FUNCTION "FC_PROG_WD" : VOID
TITLE =WORK DECKS
VERSION : 0.1


VAR_TEMP
  WD1_TEMP_IN_RANGE : BOOL ;
  WD2_TEMP_IN_RANGE : BOOL ;
  WD1_F_UP_PURGING_SP : S5TIME ;
  WD2_F_UP_PURGING_SP : S5TIME ;
  T_81CLT81_COOL_SWP : REAL ;
  T_81CLT81_HEAT_SWP : REAL ;
  T_82CLT81_COOL_SWP : REAL ;
  T_82CLT81_HEAT_SWP : REAL ;
  T_81CLT81_READY_LOW : REAL ;
  T_81CLT81_READY_HIGH : REAL ;
  T_82CLT81_READY_LOW : REAL ;
  T_82CLT81_READY_HIGH : REAL ;
END_VAR
BEGIN
NETWORK
TITLE =SET MODE WORK DECKS 1+2 ON
//
//************************* SET MODE OF WORK DECK'S ******************************
//
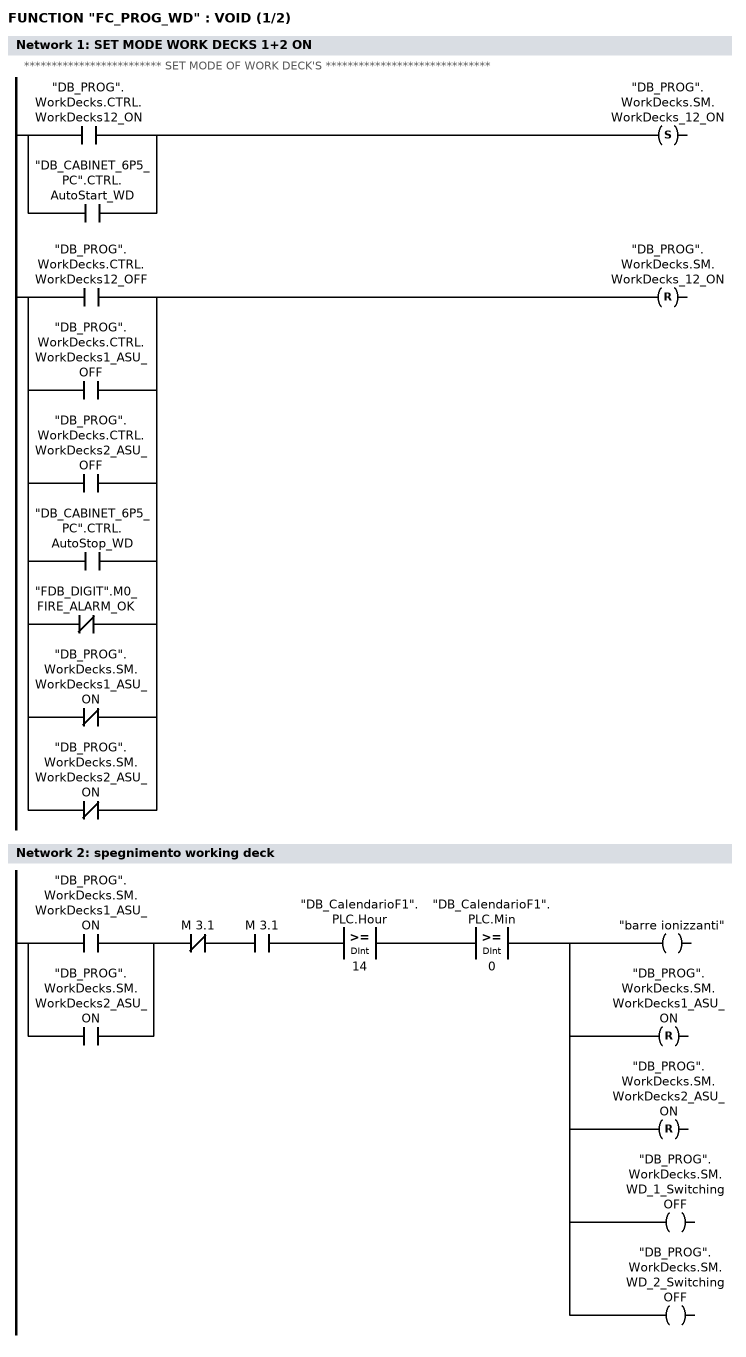
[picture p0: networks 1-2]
      U(    ;
      O     "DB_PROG".WorkDecks.CTRL.WorkDecks12_ON;
      O     "DB_CABINET_6P5_PC".CTRL.AutoStart_WD;
      )     ;
      S     "DB_PROG".WorkDecks.SM.WorkDecks_12_ON;
      U(    ;
      O     "DB_PROG".WorkDecks.CTRL.WorkDecks12_OFF;
      O     "DB_PROG".WorkDecks.CTRL.WorkDecks1_ASU_OFF;
      O     "DB_PROG".WorkDecks.CTRL.WorkDecks2_ASU_OFF;
      O     "DB_CABINET_6P5_PC".CTRL.AutoStop_WD;
      ON    "FDB_DIGIT".M0_FIRE_ALARM_OK;
      ON    "DB_PROG".WorkDecks.SM.WorkDecks1_ASU_ON;
      ON    "DB_PROG".WorkDecks.SM.WorkDecks2_ASU_ON;
      )     ;
      R     "DB_PROG".WorkDecks.SM.WorkDecks_12_ON;
      NOP   0;
NETWORK
TITLE =spegnimento working deck

      U(    ;
      O     "DB_PROG".WorkDecks.SM.WorkDecks1_ASU_ON;
      O     "DB_PROG".WorkDecks.SM.WorkDecks2_ASU_ON;
      )     ;
      UN    M      3.1;
      U     M      3.1;
      U(    ;
      L     "DB_CalendarioF1".PLC.Hour;
      L     14;
      >=D   ;
      )     ;
      U(    ;
      L     "DB_CalendarioF1".PLC.Min;
      L     0;
      >=D   ;
      )     ;
      =     "barre ionizzanti";
      R     "DB_PROG".WorkDecks.SM.WorkDecks1_ASU_ON;
      R     "DB_PROG".WorkDecks.SM.WorkDecks2_ASU_ON;
      =     "DB_PROG".WorkDecks.SM.WD_1_SwitchingOFF;
      =     "DB_PROG".WorkDecks.SM.WD_2_SwitchingOFF;
NETWORK
TITLE =SET MODE WORK DECKS 1 ON
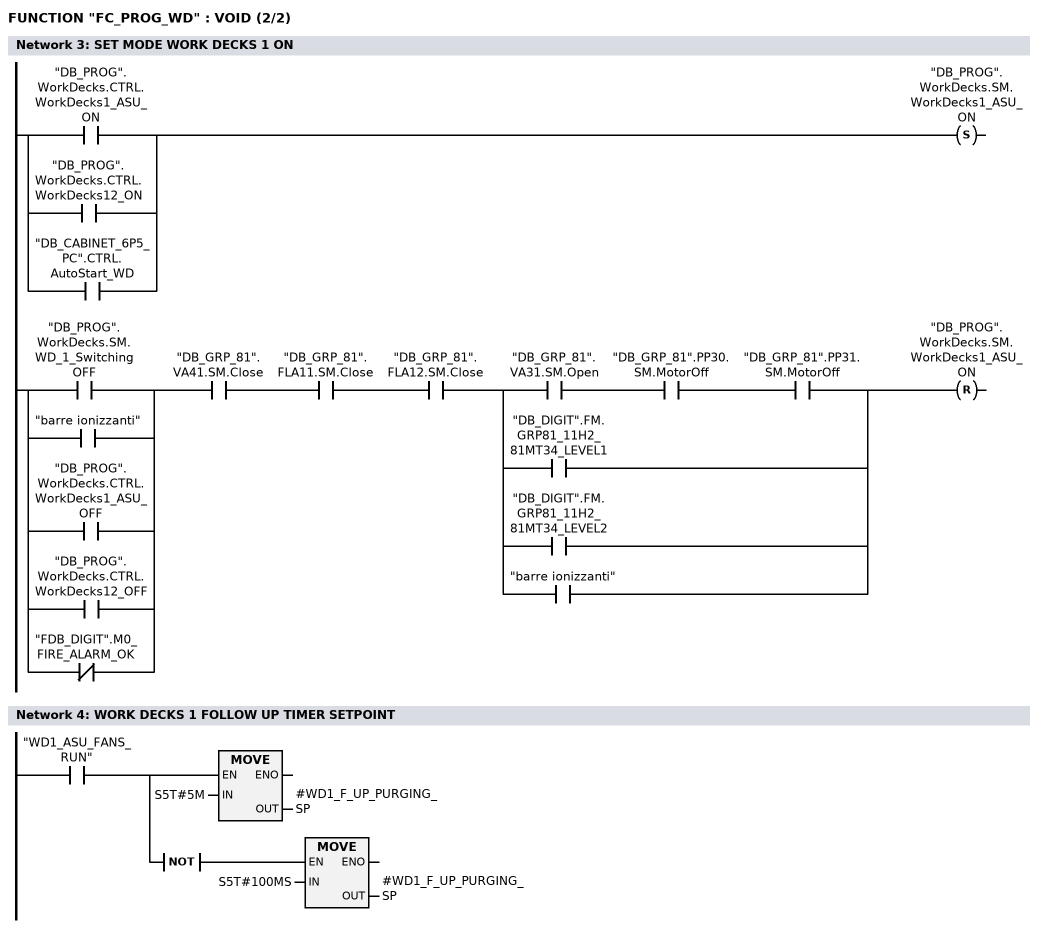
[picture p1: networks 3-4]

      U(    ;
      O     "DB_PROG".WorkDecks.CTRL.WorkDecks1_ASU_ON;
      O     "DB_PROG".WorkDecks.CTRL.WorkDecks12_ON;
      O     "DB_CABINET_6P5_PC".CTRL.AutoStart_WD;
      )     ;
      S     "DB_PROG".WorkDecks.SM.WorkDecks1_ASU_ON;
      U(    ;
      O     "DB_PROG".WorkDecks.SM.WD_1_SwitchingOFF;
      O     "barre ionizzanti";
      O     "DB_PROG".WorkDecks.CTRL.WorkDecks1_ASU_OFF;
      O     "DB_PROG".WorkDecks.CTRL.WorkDecks12_OFF;
      ON    "FDB_DIGIT".M0_FIRE_ALARM_OK;
      )     ;
      U     "DB_GRP_81".VA41.SM.Close;
      U     "DB_GRP_81".FLA11.SM.Close;
      U     "DB_GRP_81".FLA12.SM.Close;
      U(    ;
      U     "DB_GRP_81".VA31.SM.Open;
      U     "DB_GRP_81".PP30.SM.MotorOff;
      U     "DB_GRP_81".PP31.SM.MotorOff;
      O     "DB_DIGIT".FM.GRP81_11H2_81MT34_LEVEL1;
      O     "DB_DIGIT".FM.GRP81_11H2_81MT34_LEVEL2;
      O     "barre ionizzanti";
      )     ;
      R     "DB_PROG".WorkDecks.SM.WorkDecks1_ASU_ON;
      NOP   0;
NETWORK
TITLE =WORK DECKS 1 FOLLOW UP TIMER SETPOINT

      U     "WD1_ASU_FANS_RUN";
      =     L     38.0;
      U     L     38.0;
      SPBNB _001;
      L     S5T#5M;
      T     #WD1_F_UP_PURGING_SP;
_001: NOP   0;
      U     L     38.0;
      NOT   ;
      SPBNB _002;
      L     S5T#100MS;
      T     #WD1_F_UP_PURGING_SP;
_002: NOP   0;
NETWORK
TITLE =SET MODE WORK DECKS 1 SWITCHING OFF
//
//
      U(    ;
      U(    ;
      O     "DB_PROG".WorkDecks.CTRL.WorkDecks1_ASU_OFF;
      O     "barre ionizzanti";
      ON    "DB_PROG".WorkDecks.SM.WorkDecks_12_ON;
      ON    "FDB_DIGIT".M0_FIRE_ALARM_OK;
      )     ;
      U     "DB_CABINET_6P5_R11".SM.CtrlVoltageON;
      S     "DB_PROG".WorkDecks.SM.WD_1_SwitchingOFF;
      U(    ;
      U     "DB_GRP_81".VA41.SM.Close;
      U     "DB_GRP_81".FLA11.SM.Close;
      U     "DB_GRP_81".FLA12.SM.Close;
      U(    ;
      U     "DB_GRP_81".VA31.SM.Open;
      U     "DB_GRP_81".PP30.SM.MotorOff;
      U     "DB_GRP_81".PP31.SM.MotorOff;
      O     "DB_DIGIT".FM.GRP81_11H2_81MT34_LEVEL1;
      O     "DB_DIGIT".FM.GRP81_11H2_81MT34_LEVEL2;
      )     ;
      O     "DB_PROG".WorkDecks.CTRL.WorkDecks1_ASU_ON;
      O     "DB_PROG".WorkDecks.SM.WorkDecks_12_ON;
      )     ;
      R     "DB_PROG".WorkDecks.SM.WD_1_SwitchingOFF;
      U     "DB_PROG".WorkDecks.SM.WD_1_SwitchingOFF;
      )     ;
      L     #WD1_F_UP_PURGING_SP;
      SE    "T_FOLLOW_UP_PURGING_WD1";
      U(    ;
      O     "DB_PROG".WorkDecks.CTRL.WorkDecks1_ASU_ON;
      O     "DB_PROG".WorkDecks.SM.WorkDecks_12_ON;
      )     ;
      R     "T_FOLLOW_UP_PURGING_WD1";
      NOP   0;
      NOP   0;
      NOP   0;
NETWORK
TITLE =SET MODE WORK DECKS 2 ON
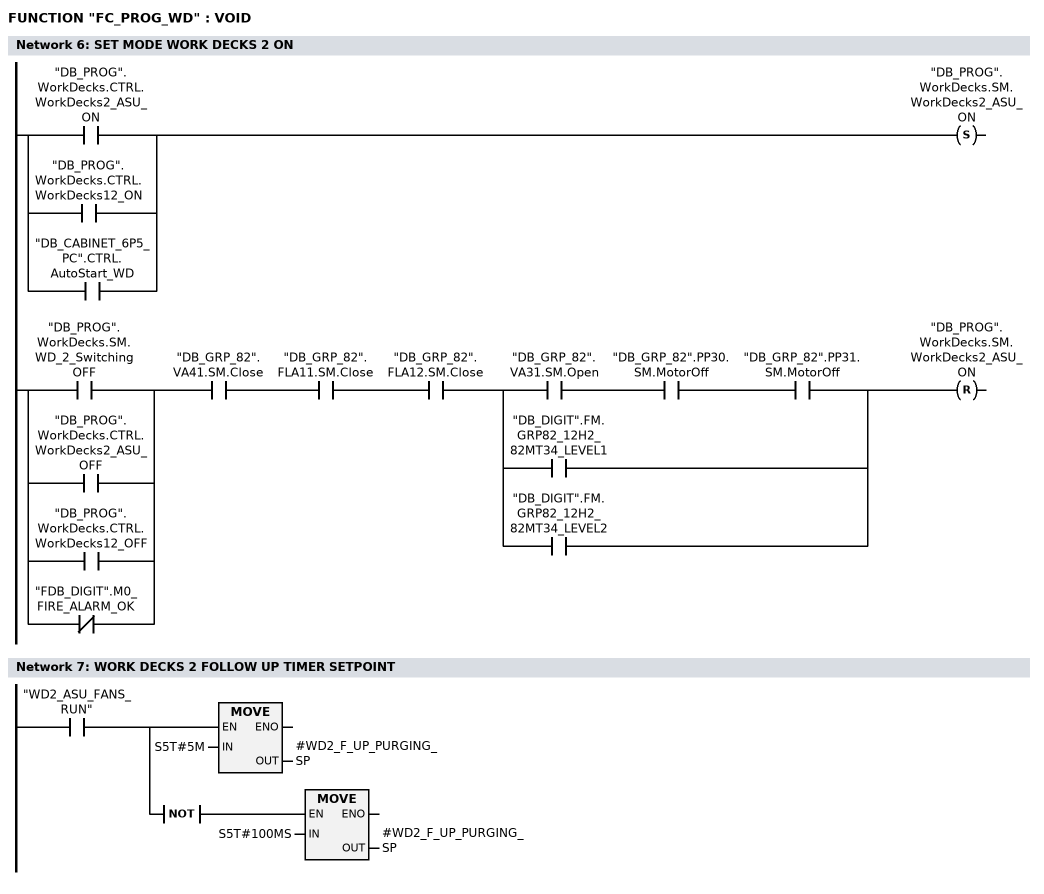
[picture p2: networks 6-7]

      U(    ;
      O     "DB_PROG".WorkDecks.CTRL.WorkDecks2_ASU_ON;
      O     "DB_PROG".WorkDecks.CTRL.WorkDecks12_ON;
      O     "DB_CABINET_6P5_PC".CTRL.AutoStart_WD;
      )     ;
      S     "DB_PROG".WorkDecks.SM.WorkDecks2_ASU_ON;
      U(    ;
      O     "DB_PROG".WorkDecks.SM.WD_2_SwitchingOFF;
      O     "DB_PROG".WorkDecks.CTRL.WorkDecks2_ASU_OFF;
      O     "DB_PROG".WorkDecks.CTRL.WorkDecks12_OFF;
      ON    "FDB_DIGIT".M0_FIRE_ALARM_OK;
      )     ;
      U     "DB_GRP_82".VA41.SM.Close;
      U     "DB_GRP_82".FLA11.SM.Close;
      U     "DB_GRP_82".FLA12.SM.Close;
      U(    ;
      U     "DB_GRP_82".VA31.SM.Open;
      U     "DB_GRP_82".PP30.SM.MotorOff;
      U     "DB_GRP_82".PP31.SM.MotorOff;
      O     "DB_DIGIT".FM.GRP82_12H2_82MT34_LEVEL1;
      O     "DB_DIGIT".FM.GRP82_12H2_82MT34_LEVEL2;
      )     ;
      R     "DB_PROG".WorkDecks.SM.WorkDecks2_ASU_ON;
      NOP   0;
NETWORK
TITLE =WORK DECKS 2 FOLLOW UP TIMER SETPOINT

      U     "WD2_ASU_FANS_RUN";
      =     L     38.0;
      U     L     38.0;
      SPBNB _003;
      L     S5T#5M;
      T     #WD2_F_UP_PURGING_SP;
_003: NOP   0;
      U     L     38.0;
      NOT   ;
      SPBNB _004;
      L     S5T#100MS;
      T     #WD2_F_UP_PURGING_SP;
_004: NOP   0;
NETWORK
TITLE =SET MODE WORK DECKS 2 SWITCHING OFF

      U(    ;
      U(    ;
      O     "DB_PROG".WorkDecks.CTRL.WorkDecks2_ASU_OFF;
      ON    "DB_PROG".WorkDecks.SM.WorkDecks_12_ON;
      ON    "FDB_DIGIT".M0_FIRE_ALARM_OK;
      )     ;
      U     "DB_CABINET_6P5_R12".SM.CtrlVoltageON;
      S     "DB_PROG".WorkDecks.SM.WD_2_SwitchingOFF;
      U(    ;
      U     "DB_GRP_82".VA41.SM.Close;
      U     "DB_GRP_82".FLA11.SM.Close;
      U     "DB_GRP_82".FLA12.SM.Close;
      U(    ;
      U     "DB_GRP_82".VA31.SM.Open;
      U     "DB_GRP_82".PP30.SM.MotorOff;
      U     "DB_GRP_82".PP31.SM.MotorOff;
      O     "DB_DIGIT".FM.GRP82_12H2_82MT34_LEVEL1;
      O     "DB_DIGIT".FM.GRP82_12H2_82MT34_LEVEL2;
      )     ;
      O     "DB_PROG".WorkDecks.CTRL.WorkDecks2_ASU_ON;
      O     "DB_PROG".WorkDecks.SM.WorkDecks_12_ON;
      )     ;
      R     "DB_PROG".WorkDecks.SM.WD_2_SwitchingOFF;
      U     "DB_PROG".WorkDecks.SM.WD_2_SwitchingOFF;
      )     ;
      L     #WD2_F_UP_PURGING_SP;
      SE    "T_FOLLOW_UP_PURGING_WD2";
      U(    ;
      O     "DB_PROG".WorkDecks.CTRL.WorkDecks2_ASU_ON;
      O     "DB_PROG".WorkDecks.SM.WorkDecks_12_ON;
      )     ;
      R     "T_FOLLOW_UP_PURGING_WD2";
      NOP   0;
      NOP   0;
      NOP   0;
NETWORK
TITLE =SET MODE VENTILATION SKID OFF-CLEANING ON
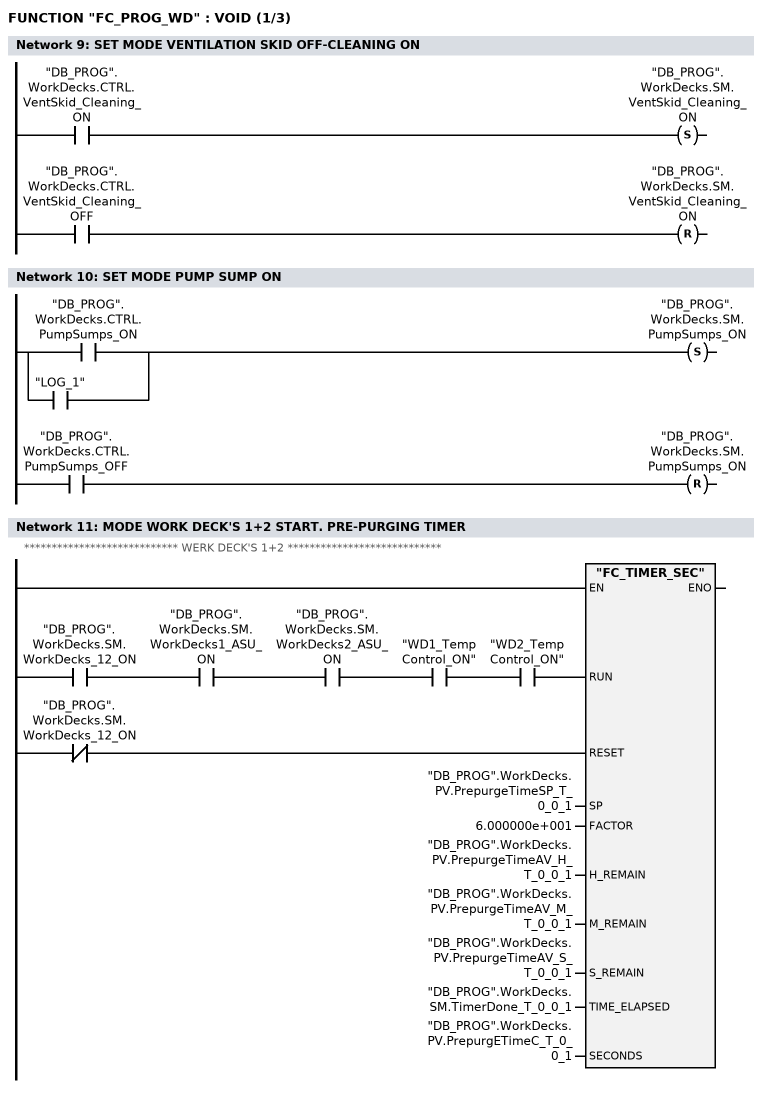
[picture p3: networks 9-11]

      U     "DB_PROG".WorkDecks.CTRL.VentSkid_Cleaning_ON;
      S     "DB_PROG".WorkDecks.SM.VentSkid_Cleaning_ON;
      U     "DB_PROG".WorkDecks.CTRL.VentSkid_Cleaning_OFF;
      R     "DB_PROG".WorkDecks.SM.VentSkid_Cleaning_ON;
      NOP   0;
NETWORK
TITLE =SET MODE PUMP SUMP ON

      U(    ;
      O     "DB_PROG".WorkDecks.CTRL.PumpSumps_ON;
      O     "LOG_1";
      )     ;
      S     "DB_PROG".WorkDecks.SM.PumpSumps_ON;
      U     "DB_PROG".WorkDecks.CTRL.PumpSumps_OFF;
      R     "DB_PROG".WorkDecks.SM.PumpSumps_ON;
      NOP   0;
NETWORK
TITLE =MODE WORK DECK'S 1+2 START. PRE-PURGING TIMER
//
//**************************** WERK DECK'S 1+2 ****************************
//
      U     "DB_PROG".WorkDecks.SM.WorkDecks_12_ON;
      U     "DB_PROG".WorkDecks.SM.WorkDecks1_ASU_ON;
      U     "DB_PROG".WorkDecks.SM.WorkDecks2_ASU_ON;
      U     "WD1_TempControl_ON";
      U     "WD2_TempControl_ON";
      =     L     38.0;
      BLD   103;
      UN    "DB_PROG".WorkDecks.SM.WorkDecks_12_ON;
      =     L     38.1;
      BLD   103;
      CALL "FC_TIMER_SEC" (
           RUN                      := L     38.0,
           RESET                    := L     38.1,
           SP                       := "DB_PROG".WorkDecks.PV.PrepurgeTimeSP_T_0_0_1,
           FACTOR                   := 6.000000e+001,
           H_REMAIN                 := "DB_PROG".WorkDecks.PV.PrepurgeTimeAV_H_T_0_0_1,
           M_REMAIN                 := "DB_PROG".WorkDecks.PV.PrepurgeTimeAV_M_T_0_0_1,
           S_REMAIN                 := "DB_PROG".WorkDecks.PV.PrepurgeTimeAV_S_T_0_0_1,
           TIME_ELAPSED             := "DB_PROG".WorkDecks.SM.TimerDone_T_0_0_1,
           SECONDS                  := "DB_PROG".WorkDecks.PV.PrepurgETimeC_T_0_0_1);
      NOP   0;
NETWORK
TITLE =MODE WORK DECK'S 1 START. PRE-PURGING TIMER
//
//**************************** WERK DECK'S 1 ****************************
//
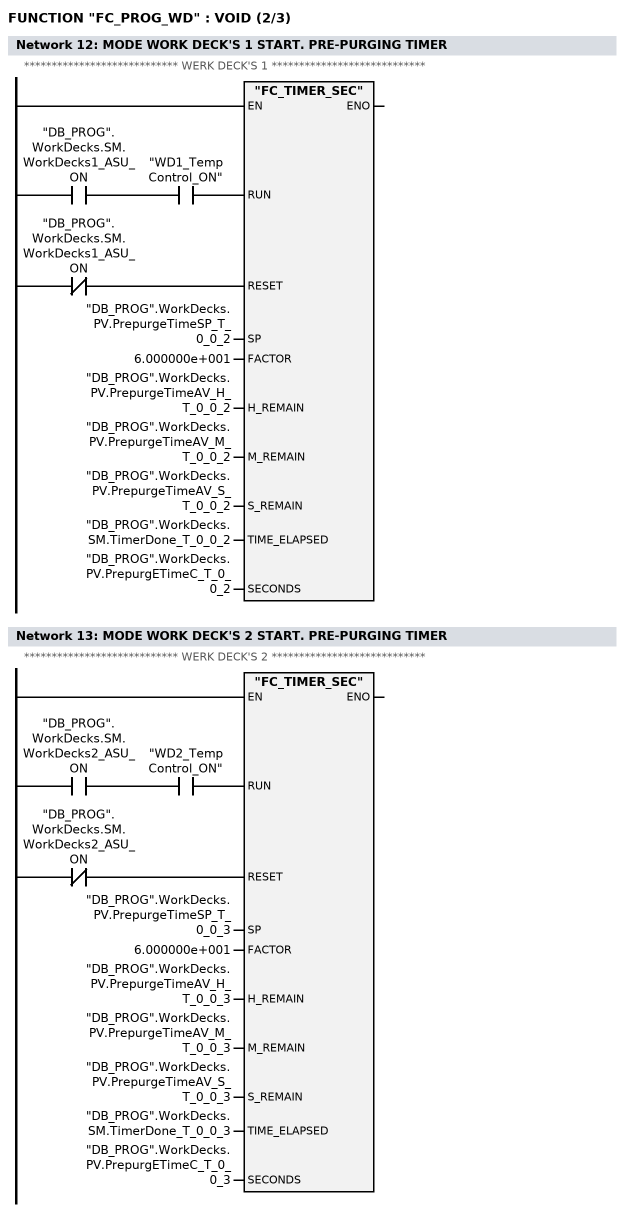
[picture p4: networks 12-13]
      U     "DB_PROG".WorkDecks.SM.WorkDecks1_ASU_ON;
      U     "WD1_TempControl_ON";
      =     L     38.0;
      BLD   103;
      UN    "DB_PROG".WorkDecks.SM.WorkDecks1_ASU_ON;
      =     L     38.1;
      BLD   103;
      CALL "FC_TIMER_SEC" (
           RUN                      := L     38.0,
           RESET                    := L     38.1,
           SP                       := "DB_PROG".WorkDecks.PV.PrepurgeTimeSP_T_0_0_2,
           FACTOR                   := 6.000000e+001,
           H_REMAIN                 := "DB_PROG".WorkDecks.PV.PrepurgeTimeAV_H_T_0_0_2,
           M_REMAIN                 := "DB_PROG".WorkDecks.PV.PrepurgeTimeAV_M_T_0_0_2,
           S_REMAIN                 := "DB_PROG".WorkDecks.PV.PrepurgeTimeAV_S_T_0_0_2,
           TIME_ELAPSED             := "DB_PROG".WorkDecks.SM.TimerDone_T_0_0_2,
           SECONDS                  := "DB_PROG".WorkDecks.PV.PrepurgETimeC_T_0_0_2);
      NOP   0;
NETWORK
TITLE =MODE WORK DECK'S 2 START. PRE-PURGING TIMER
//
//**************************** WERK DECK'S 2 ****************************
//
      U     "DB_PROG".WorkDecks.SM.WorkDecks2_ASU_ON;
      U     "WD2_TempControl_ON";
      =     L     38.0;
      BLD   103;
      UN    "DB_PROG".WorkDecks.SM.WorkDecks2_ASU_ON;
      =     L     38.1;
      BLD   103;
      CALL "FC_TIMER_SEC" (
           RUN                      := L     38.0,
           RESET                    := L     38.1,
           SP                       := "DB_PROG".WorkDecks.PV.PrepurgeTimeSP_T_0_0_3,
           FACTOR                   := 6.000000e+001,
           H_REMAIN                 := "DB_PROG".WorkDecks.PV.PrepurgeTimeAV_H_T_0_0_3,
           M_REMAIN                 := "DB_PROG".WorkDecks.PV.PrepurgeTimeAV_M_T_0_0_3,
           S_REMAIN                 := "DB_PROG".WorkDecks.PV.PrepurgeTimeAV_S_T_0_0_3,
           TIME_ELAPSED             := "DB_PROG".WorkDecks.SM.TimerDone_T_0_0_3,
           SECONDS                  := "DB_PROG".WorkDecks.PV.PrepurgETimeC_T_0_0_3);
      NOP   0;
NETWORK
TITLE =MODE WORK DECK'S OFF-LINE SKID CLEANING START. PRE-PURGING TIMER
//
//****************** WORK DECK'S OFF-LINE SKID CLEANING *******************
//
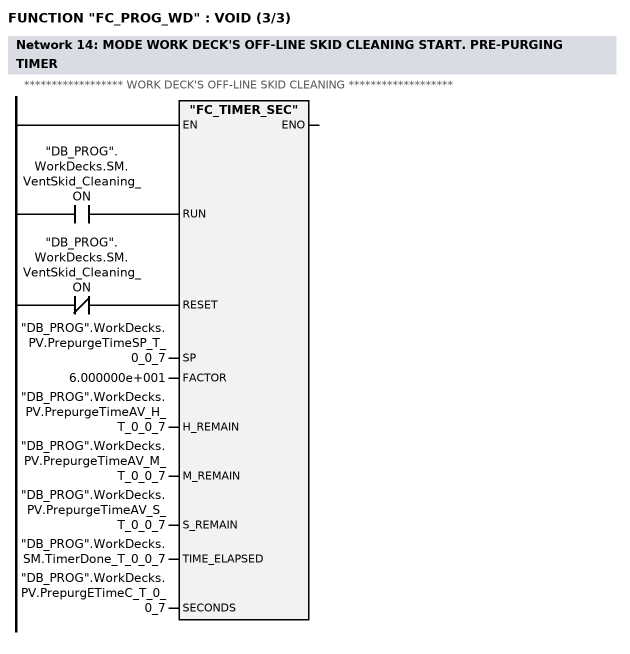
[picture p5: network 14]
      U     "DB_PROG".WorkDecks.SM.VentSkid_Cleaning_ON;
      =     L     38.0;
      BLD   103;
      UN    "DB_PROG".WorkDecks.SM.VentSkid_Cleaning_ON;
      =     L     38.1;
      BLD   103;
      CALL "FC_TIMER_SEC" (
           RUN                      := L     38.0,
           RESET                    := L     38.1,
           SP                       := "DB_PROG".WorkDecks.PV.PrepurgeTimeSP_T_0_0_7,
           FACTOR                   := 6.000000e+001,
           H_REMAIN                 := "DB_PROG".WorkDecks.PV.PrepurgeTimeAV_H_T_0_0_7,
           M_REMAIN                 := "DB_PROG".WorkDecks.PV.PrepurgeTimeAV_M_T_0_0_7,
           S_REMAIN                 := "DB_PROG".WorkDecks.PV.PrepurgeTimeAV_S_T_0_0_7,
           TIME_ELAPSED             := "DB_PROG".WorkDecks.SM.TimerDone_T_0_0_7,
           SECONDS                  := "DB_PROG".WorkDecks.PV.PrepurgETimeC_T_0_0_7);
      NOP   0;
NETWORK
TITLE =MODE START WORK DECK'S 1
//
//**************** START SEQUENTION WORK DECK'S 1 ******************************
//
      U(    ;
      U(    ;
      O     "DB_PROG".WorkDecks.CTRL.WorkDecks1_ASU_ON;
      O     "DB_PROG".WorkDecks.SM.WorkDecks_12_ON;
      )     ;
      S     "WD1_ASU_StartPump";
      U     "WD1_StartFinished";
      R     "WD1_ASU_StartPump";
      U     "WD1_ASU_StartPump";
      )     ;
      L     S5T#5M;
      SE    "T_2_0_10";
      NOP   0;
      NOP   0;
      NOP   0;
      NOP   0;
NETWORK
TITLE =WORK DECKS #1 DELAY STOP PUMP =81PP31 ASU WD1, WHEN TEMP>TEMP_SP
//
//
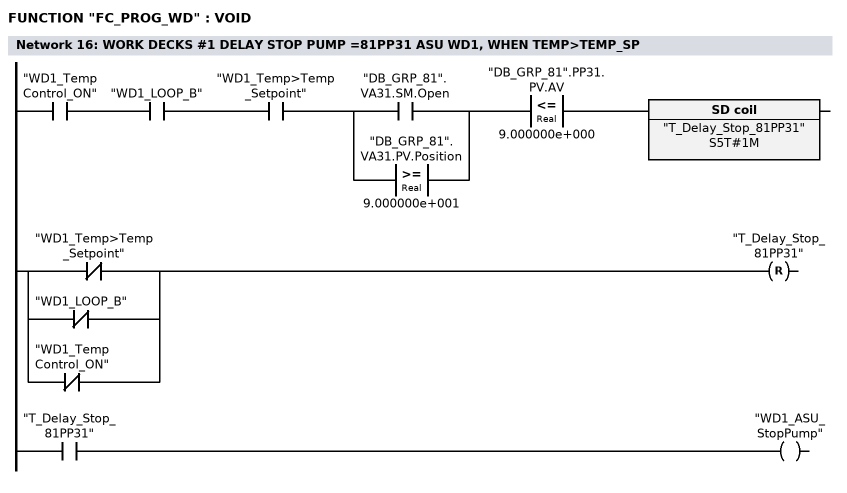
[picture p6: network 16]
      U     "WD1_TempControl_ON";
      U     "WD1_LOOP_B";
      U     "WD1_Temp>Temp_Setpoint";
      U(    ;
      O     "DB_GRP_81".VA31.SM.Open;
      O(    ;
      L     "DB_GRP_81".VA31.PV.Position;
      L     9.000000e+001;
      >=R   ;
      )     ;
      )     ;
      U(    ;
      L     "DB_GRP_81".PP31.PV.AV;
      L     9.000000e+000;
      <=R   ;
      )     ;
      L     S5T#1M;
      SE    "T_Delay_Stop_81PP31";
      U(    ;
      ON    "WD1_Temp>Temp_Setpoint";
      ON    "WD1_LOOP_B";
      ON    "WD1_TempControl_ON";
      )     ;
      R     "T_Delay_Stop_81PP31";
      NOP   0;
      NOP   0;
      U     "T_Delay_Stop_81PP31";
      =     "WD1_ASU_StopPump";
NETWORK
TITLE =START FLAPS ASU WD 1

      U     "DB_PROG".WorkDecks.SM.WorkDecks1_ASU_ON;
      U(    ;
      O     "T_2_0_10";
      O     "WD1_StartFinished";
      )     ;
      UN    "DB_MULFUNCTION".SM.WD1_MALFUNCTION_STOP;
      S     "WD1_OpenFlaps";
      U(    ;
      U(    ;
      U     "DB_PROG".WorkDecks.SM.WD_1_SwitchingOFF;
      U     "DB_GRP_81".FAN71.SM.MotorOff;
      U(    ;
      U     "DB_GRP_81".FAN01.SM.MotorOff;
      U     "DB_GRP_82".FAN02.SM.MotorOff;
      ON    "DB_PROG".WorkDecks.SM.WorkDecks_12_ON;
      )     ;
      O     "DB_DIGIT".FM.GRP81_11H2_81MT34_LEVEL2;
      )     ;
      L     S5T#3M;
      SE    "T_5_0_2";
      NOP   0;
      NOP   0;
      NOP   0;
      U     "T_5_0_2";
      )     ;
      R     "WD1_OpenFlaps";
      NOP   0;
NETWORK
TITLE =VENTILATION WORK DECK'S 1 RUNNING (SIGNAL TO SHOP)
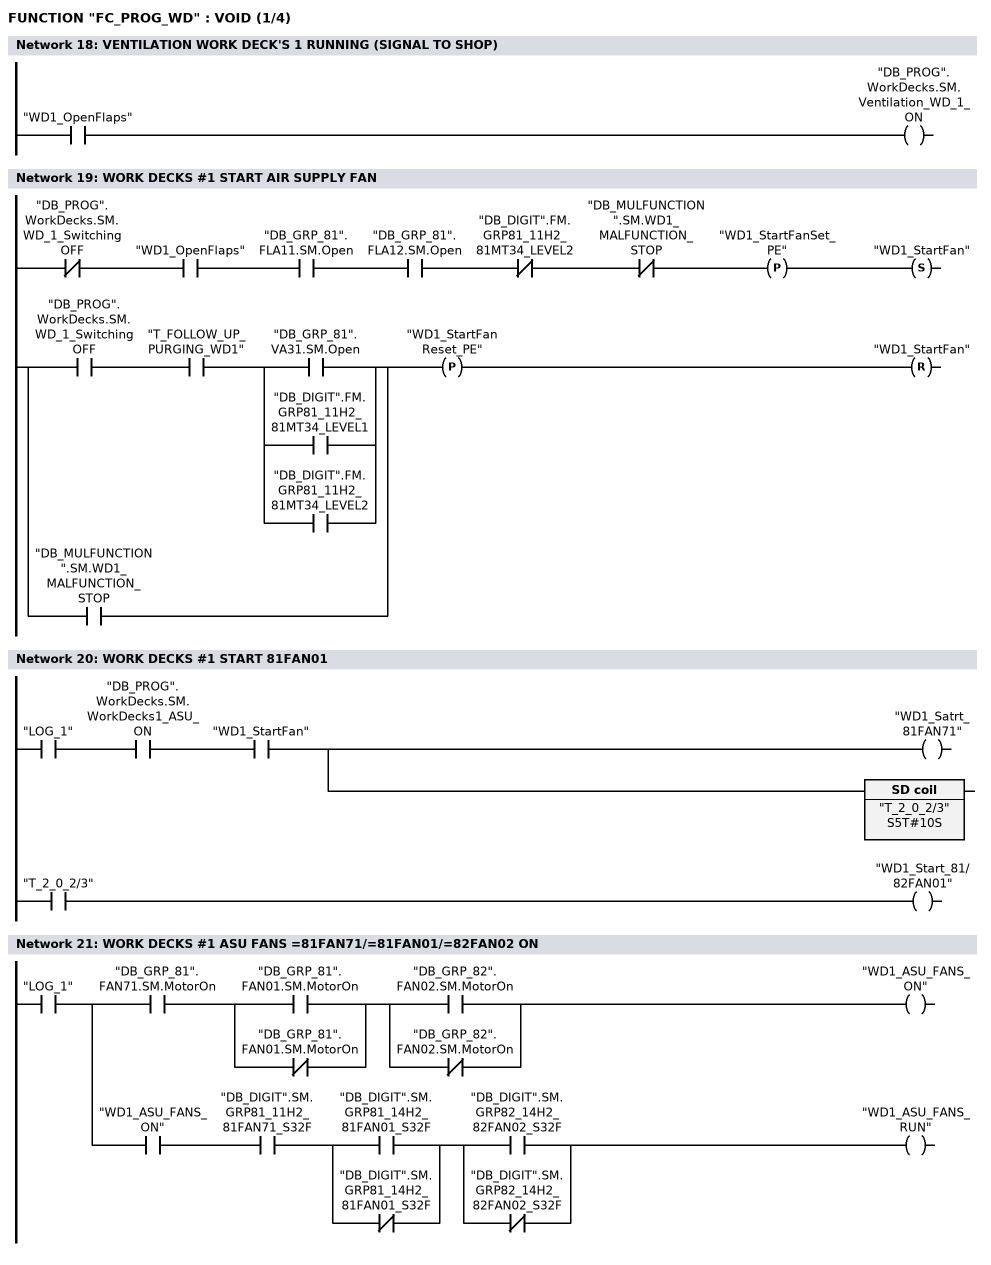
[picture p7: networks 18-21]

      U     "WD1_OpenFlaps";
      =     "DB_PROG".WorkDecks.SM.Ventilation_WD_1_ON;
NETWORK
TITLE =WORK DECKS #1 START AIR SUPPLY FAN

      UN    "DB_PROG".WorkDecks.SM.WD_1_SwitchingOFF;
      U     "WD1_OpenFlaps";
      U     "DB_GRP_81".FLA11.SM.Open;
      U     "DB_GRP_81".FLA12.SM.Open;
      UN    "DB_DIGIT".FM.GRP81_11H2_81MT34_LEVEL2;
      UN    "DB_MULFUNCTION".SM.WD1_MALFUNCTION_STOP;
      FP    "WD1_StartFanSet_PE";
      S     "WD1_StartFan";
      U(    ;
      U     "DB_PROG".WorkDecks.SM.WD_1_SwitchingOFF;
      U     "T_FOLLOW_UP_PURGING_WD1";
      U(    ;
      O     "DB_GRP_81".VA31.SM.Open;
      O     "DB_DIGIT".FM.GRP81_11H2_81MT34_LEVEL1;
      O     "DB_DIGIT".FM.GRP81_11H2_81MT34_LEVEL2;
      )     ;
      O     "DB_MULFUNCTION".SM.WD1_MALFUNCTION_STOP;
      )     ;
      FP    "WD1_StartFanReset_PE";
      R     "WD1_StartFan";
      NOP   0;
NETWORK
TITLE =WORK DECKS #1 START 81FAN01

      U     "LOG_1";
      U     "DB_PROG".WorkDecks.SM.WorkDecks1_ASU_ON;
      U     "WD1_StartFan";
      =     L     38.0;
      U     L     38.0;
      BLD   102;
      =     "WD1_Satrt_81FAN71";
      U     L     38.0;
      L     S5T#10S;
      SE    "T_2_0_2/3";
      NOP   0;
      NOP   0;
      NOP   0;
      U     "T_2_0_2/3";
      =     "WD1_Start_81/82FAN01";
NETWORK
TITLE =WORK DECKS #1 ASU FANS =81FAN71/=81FAN01/=82FAN02 ON

      U     "LOG_1";
      =     L     38.0;
      U     L     38.0;
      U     "DB_GRP_81".FAN71.SM.MotorOn;
      U(    ;
      O     "DB_GRP_81".FAN01.SM.MotorOn;
      ON    "DB_GRP_81".FAN01.SM.MotorOn;
      )     ;
      U(    ;
      O     "DB_GRP_82".FAN02.SM.MotorOn;
      ON    "DB_GRP_82".FAN02.SM.MotorOn;
      )     ;
      =     "WD1_ASU_FANS_ON";
      U     L     38.0;
      U     "WD1_ASU_FANS_ON";
      U     "DB_DIGIT".SM.GRP81_11H2_81FAN71_S32F;
      U(    ;
      O     "DB_DIGIT".SM.GRP81_14H2_81FAN01_S32F;
      ON    "DB_DIGIT".SM.GRP81_14H2_81FAN01_S32F;
      )     ;
      U(    ;
      O     "DB_DIGIT".SM.GRP82_14H2_82FAN02_S32F;
      ON    "DB_DIGIT".SM.GRP82_14H2_82FAN02_S32F;
      )     ;
      =     "WD1_ASU_FANS_RUN";
NETWORK
TITLE =WORK DECKS #1 TEMPERATURE CONTROL ON (PAP 1.5.1)
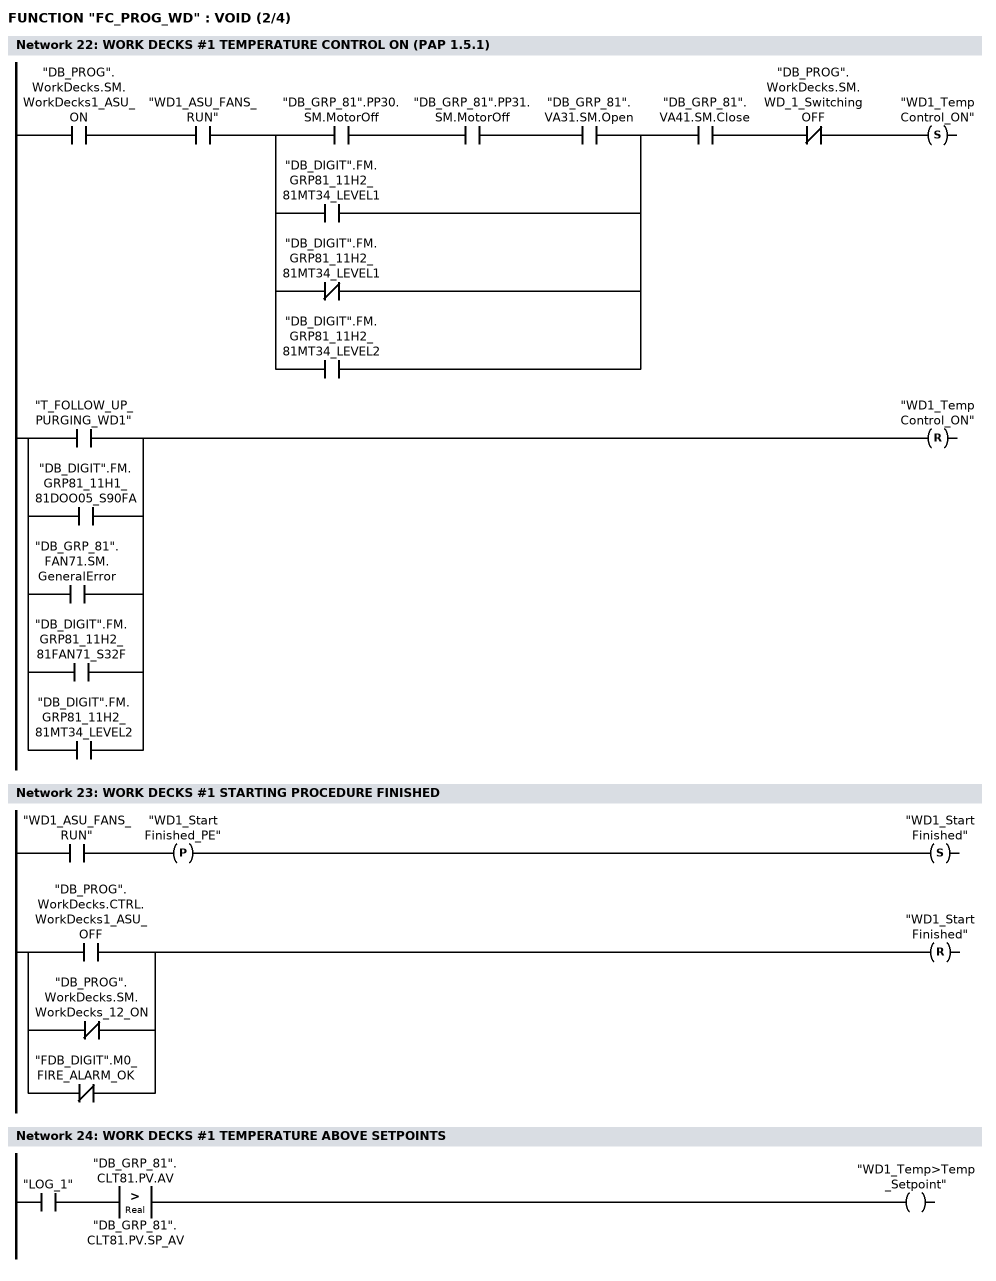
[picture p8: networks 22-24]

      U     "DB_PROG".WorkDecks.SM.WorkDecks1_ASU_ON;
      U     "WD1_ASU_FANS_RUN";
      U(    ;
      U     "DB_GRP_81".PP30.SM.MotorOff;
      U     "DB_GRP_81".PP31.SM.MotorOff;
      U     "DB_GRP_81".VA31.SM.Open;
      O     "DB_DIGIT".FM.GRP81_11H2_81MT34_LEVEL1;
      ON    "DB_DIGIT".FM.GRP81_11H2_81MT34_LEVEL1;
      O     "DB_DIGIT".FM.GRP81_11H2_81MT34_LEVEL2;
      )     ;
      U     "DB_GRP_81".VA41.SM.Close;
      UN    "DB_PROG".WorkDecks.SM.WD_1_SwitchingOFF;
      S     "WD1_TempControl_ON";
      U(    ;
      O     "T_FOLLOW_UP_PURGING_WD1";
      O     "DB_DIGIT".FM.GRP81_11H1_81DOO05_S90FA;
      O     "DB_GRP_81".FAN71.SM.GeneralError;
      O     "DB_DIGIT".FM.GRP81_11H2_81FAN71_S32F;
      O     "DB_DIGIT".FM.GRP81_11H2_81MT34_LEVEL2;
      )     ;
      R     "WD1_TempControl_ON";
      NOP   0;
NETWORK
TITLE =WORK DECKS #1 STARTING PROCEDURE FINISHED

      U     "WD1_ASU_FANS_RUN";
      FP    "WD1_StartFinished_PE";
      S     "WD1_StartFinished";
      U(    ;
      O     "DB_PROG".WorkDecks.CTRL.WorkDecks1_ASU_OFF;
      ON    "DB_PROG".WorkDecks.SM.WorkDecks_12_ON;
      ON    "FDB_DIGIT".M0_FIRE_ALARM_OK;
      )     ;
      R     "WD1_StartFinished";
      NOP   0;
NETWORK
TITLE =WORK DECKS #1 TEMPERATURE ABOVE SETPOINTS

      U     "LOG_1";
      U(    ;
      L     "DB_GRP_81".CLT81.PV.AV;
      L     "DB_GRP_81".CLT81.PV.SP_AV;
      >R    ;
      )     ;
      =     "WD1_Temp>Temp_Setpoint";
NETWORK
TITLE =WORK DECKS #1 SET SWITCHING POINTS
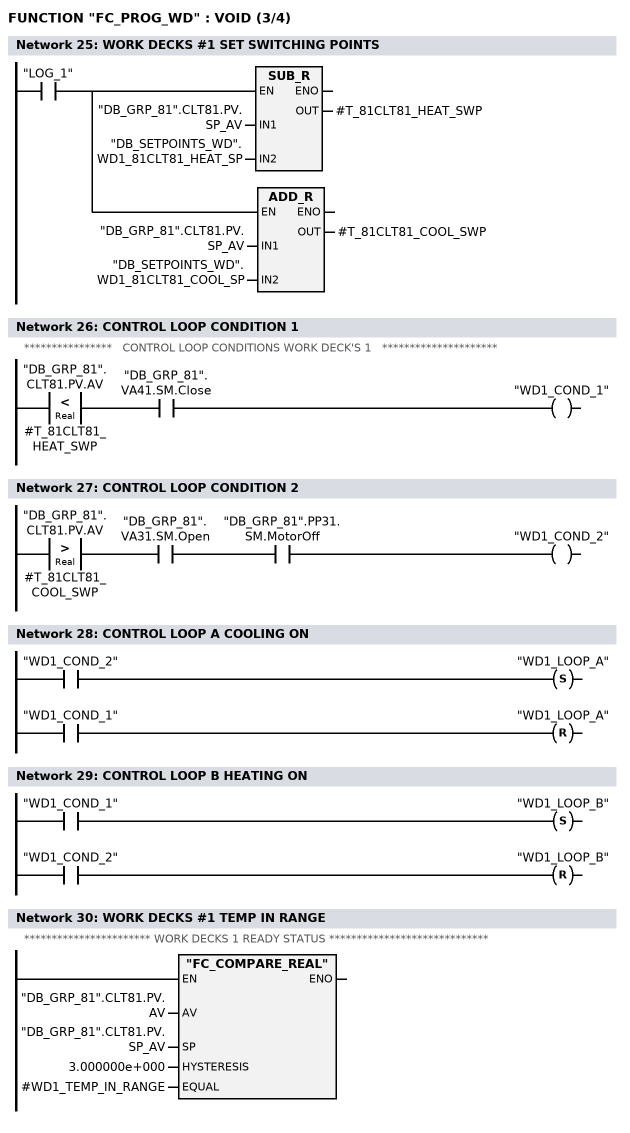
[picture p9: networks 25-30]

      U     "LOG_1";
      =     L     38.0;
      U     L     38.0;
      SPBNB _005;
      L     "DB_GRP_81".CLT81.PV.SP_AV;
      L     "DB_SETPOINTS_WD".WD1_81CLT81_HEAT_SP;
      -R    ;
      T     #T_81CLT81_HEAT_SWP;
_005: NOP   0;
      U     L     38.0;
      SPBNB _006;
      L     "DB_GRP_81".CLT81.PV.SP_AV;
      L     "DB_SETPOINTS_WD".WD1_81CLT81_COOL_SP;
      +R    ;
      T     #T_81CLT81_COOL_SWP;
_006: NOP   0;
NETWORK
TITLE =CONTROL LOOP CONDITION 1
//
//****************   CONTROL LOOP CONDITIONS WORK DECK'S 1   *********************
//
//
      U(    ;
      L     "DB_GRP_81".CLT81.PV.AV;
      L     #T_81CLT81_HEAT_SWP;
      <R    ;
      )     ;
      U     "DB_GRP_81".VA41.SM.Close;
      =     "WD1_COND_1";
NETWORK
TITLE =CONTROL LOOP CONDITION 2

      U(    ;
      L     "DB_GRP_81".CLT81.PV.AV;
      L     #T_81CLT81_COOL_SWP;
      >R    ;
      )     ;
      U     "DB_GRP_81".VA31.SM.Open;
      U     "DB_GRP_81".PP31.SM.MotorOff;
      =     "WD1_COND_2";
NETWORK
TITLE =CONTROL LOOP A COOLING ON

      U     "WD1_COND_2";
      S     "WD1_LOOP_A";
      U     "WD1_COND_1";
      R     "WD1_LOOP_A";
      NOP   0;
NETWORK
TITLE =CONTROL LOOP B HEATING ON

      U     "WD1_COND_1";
      S     "WD1_LOOP_B";
      U     "WD1_COND_2";
      R     "WD1_LOOP_B";
      NOP   0;
NETWORK
TITLE =WORK DECKS #1 TEMP IN RANGE
//
//*********************** WORK DECKS 1 READY STATUS *****************************
//
      CALL "FC_COMPARE_REAL" (
           AV                       := "DB_GRP_81".CLT81.PV.AV,
           SP                       := "DB_GRP_81".CLT81.PV.SP_AV,
           HYSTERESIS               := 3.000000e+000,
           EQUAL                    := #WD1_TEMP_IN_RANGE);
      NOP   0;
NETWORK
TITLE =WORK DECKS #1 WINDOW TO READY STATUS IN POWER SAVING MODE 2
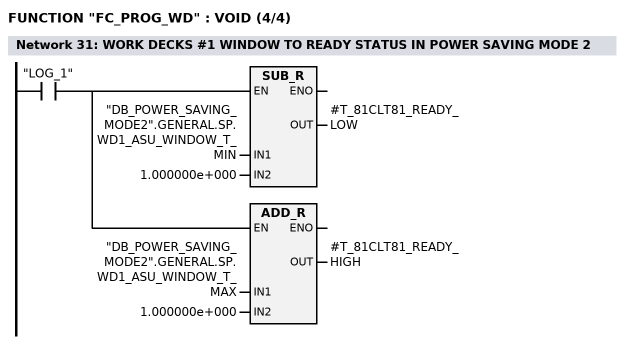
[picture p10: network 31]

      U     "LOG_1";
      =     L     38.0;
      U     L     38.0;
      SPBNB _007;
      L     "DB_POWER_SAVING_MODE2".GENERAL.SP.WD1_ASU_WINDOW_T_MIN;
      L     1.000000e+000;
      -R    ;
      T     #T_81CLT81_READY_LOW;
_007: NOP   0;
      U     L     38.0;
      SPBNB _008;
      L     "DB_POWER_SAVING_MODE2".GENERAL.SP.WD1_ASU_WINDOW_T_MAX;
      L     1.000000e+000;
      +R    ;
      T     #T_81CLT81_READY_HIGH;
_008: NOP   0;
NETWORK
TITLE =WORK DECKS #1 READY

      U(    ;
      U     "DB_PROG".WorkDecks.SM.WorkDecks1_ASU_ON;
      U(    ;
      O     "DB_PROG".WorkDecks.SM.TimerDone_T_0_0_2;
      O     "DB_PROG".WorkDecks.SM.TimerDone_T_0_0_1;
      )     ;
      U(    ;
      UN    "DB_POWER_SAVING_MODE2".GENERAL.SM.WD1_MODE_2_ON;
      U     #WD1_TEMP_IN_RANGE;
      O     ;
      U     "DB_POWER_SAVING_MODE2".GENERAL.SM.WD1_MODE_2_ON;
      U(    ;
      L     "DB_GRP_81".CLT81.PV.AV;
      L     #T_81CLT81_READY_LOW;
      >=R   ;
      )     ;
      U(    ;
      L     "DB_GRP_81".CLT81.PV.AV;
      L     #T_81CLT81_READY_HIGH;
      <=R   ;
      )     ;
      )     ;
      L     S5T#1M;
      SE    "T_WD1_READY";
      NOP   0;
      NOP   0;
      NOP   0;
      U     "T_WD1_READY";
      )     ;
      S     "DB_PROG".WorkDecks.SM.WD_1_Ready;
      U(    ;
      U(    ;
      ON    "DB_PROG".WorkDecks.SM.WorkDecks1_ASU_ON;
      O     ;
      UN    "DB_POWER_SAVING_MODE2".GENERAL.SM.WD1_MODE_2_ON;
      UN    #WD1_TEMP_IN_RANGE;
      O     ;
      U     "DB_POWER_SAVING_MODE2".GENERAL.SM.WD1_MODE_2_ON;
      U(    ;
      O(    ;
      L     "DB_GRP_81".CLT81.PV.AV;
      L     #T_81CLT81_READY_LOW;
      <R    ;
      )     ;
      O(    ;
      L     "DB_GRP_81".CLT81.PV.AV;
      L     #T_81CLT81_READY_HIGH;
      >R    ;
      )     ;
      )     ;
      )     ;
      L     S5T#1M;
      SE    "T_WD1_READY_LOST_DEL";
      NOP   0;
      NOP   0;
      NOP   0;
      U     "T_WD1_READY_LOST_DEL";
      )     ;
      R     "DB_PROG".WorkDecks.SM.WD_1_Ready;
      NOP   0;
NETWORK
TITLE =WORK DECKS #1 OPEN MANUAL CLEANING VALVES =81VA191/=82VA192

      U     "WD1_TempControl_ON";
      UN    "DB_MULFUNCTION".SM.WD1_MALFUNCTION_STOP;
      =     "WD1_OpenMClean_Flaps";
NETWORK
TITLE =MODE START WORK DECK'S 2
//
//**************** START SEQUENTION WORK DECK'S 2 ******************************
//
      U(    ;
      U(    ;
      O     "DB_PROG".WorkDecks.CTRL.WorkDecks2_ASU_ON;
      O     "DB_PROG".WorkDecks.SM.WorkDecks_12_ON;
      )     ;
      S     "WD2_ASU_StartPump";
      U     "WD2_StartFinished";
      R     "WD2_ASU_StartPump";
      U     "WD2_ASU_StartPump";
      )     ;
      L     S5T#5M;
      SE    "T_3_0_10";
      NOP   0;
      NOP   0;
      NOP   0;
      NOP   0;
NETWORK
TITLE =WORK DECKS #2 DELAY STOP PUMP =82PP31 ASU WD2, WHEN TEMP>TEMP_SP
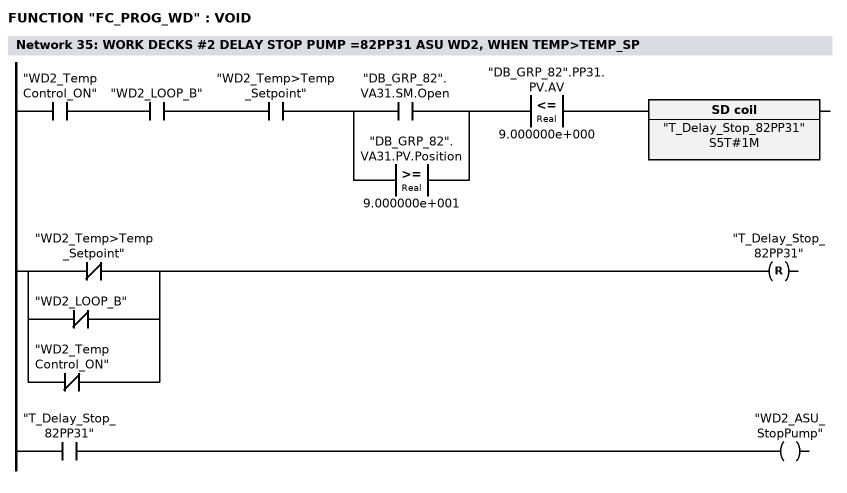
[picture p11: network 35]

      U     "WD2_TempControl_ON";
      U     "WD2_LOOP_B";
      U     "WD2_Temp>Temp_Setpoint";
      U(    ;
      O     "DB_GRP_82".VA31.SM.Open;
      O(    ;
      L     "DB_GRP_82".VA31.PV.Position;
      L     9.000000e+001;
      >=R   ;
      )     ;
      )     ;
      U(    ;
      L     "DB_GRP_82".PP31.PV.AV;
      L     9.000000e+000;
      <=R   ;
      )     ;
      L     S5T#1M;
      SE    "T_Delay_Stop_82PP31";
      U(    ;
      ON    "WD2_Temp>Temp_Setpoint";
      ON    "WD2_LOOP_B";
      ON    "WD2_TempControl_ON";
      )     ;
      R     "T_Delay_Stop_82PP31";
      NOP   0;
      NOP   0;
      U     "T_Delay_Stop_82PP31";
      =     "WD2_ASU_StopPump";
NETWORK
TITLE =START FLAPS ASU WD 2

      U     "DB_PROG".WorkDecks.SM.WorkDecks2_ASU_ON;
      U(    ;
      O     "T_3_0_10";
      O     "WD2_StartFinished";
      )     ;
      UN    "DB_MULFUNCTION".SM.WD2_MALFUNCTION_STOP;
      S     "WD2_OpenFlaps";
      U(    ;
      U(    ;
      U     "DB_PROG".WorkDecks.SM.WD_2_SwitchingOFF;
      U     "DB_GRP_82".FAN71.SM.MotorOff;
      U(    ;
      U     "DB_GRP_81".FAN01.SM.MotorOff;
      U     "DB_GRP_82".FAN02.SM.MotorOff;
      ON    "DB_PROG".WorkDecks.SM.WorkDecks_12_ON;
      )     ;
      O     "DB_DIGIT".FM.GRP82_12H2_82MT34_LEVEL2;
      )     ;
      L     S5T#3M;
      SE    "T_6_0_2";
      NOP   0;
      NOP   0;
      NOP   0;
      U     "T_6_0_2";
      )     ;
      R     "WD2_OpenFlaps";
      NOP   0;
NETWORK
TITLE =VENTILATION WORK DECK'S 2 RUNNING (SIGNAL TO SHOP)
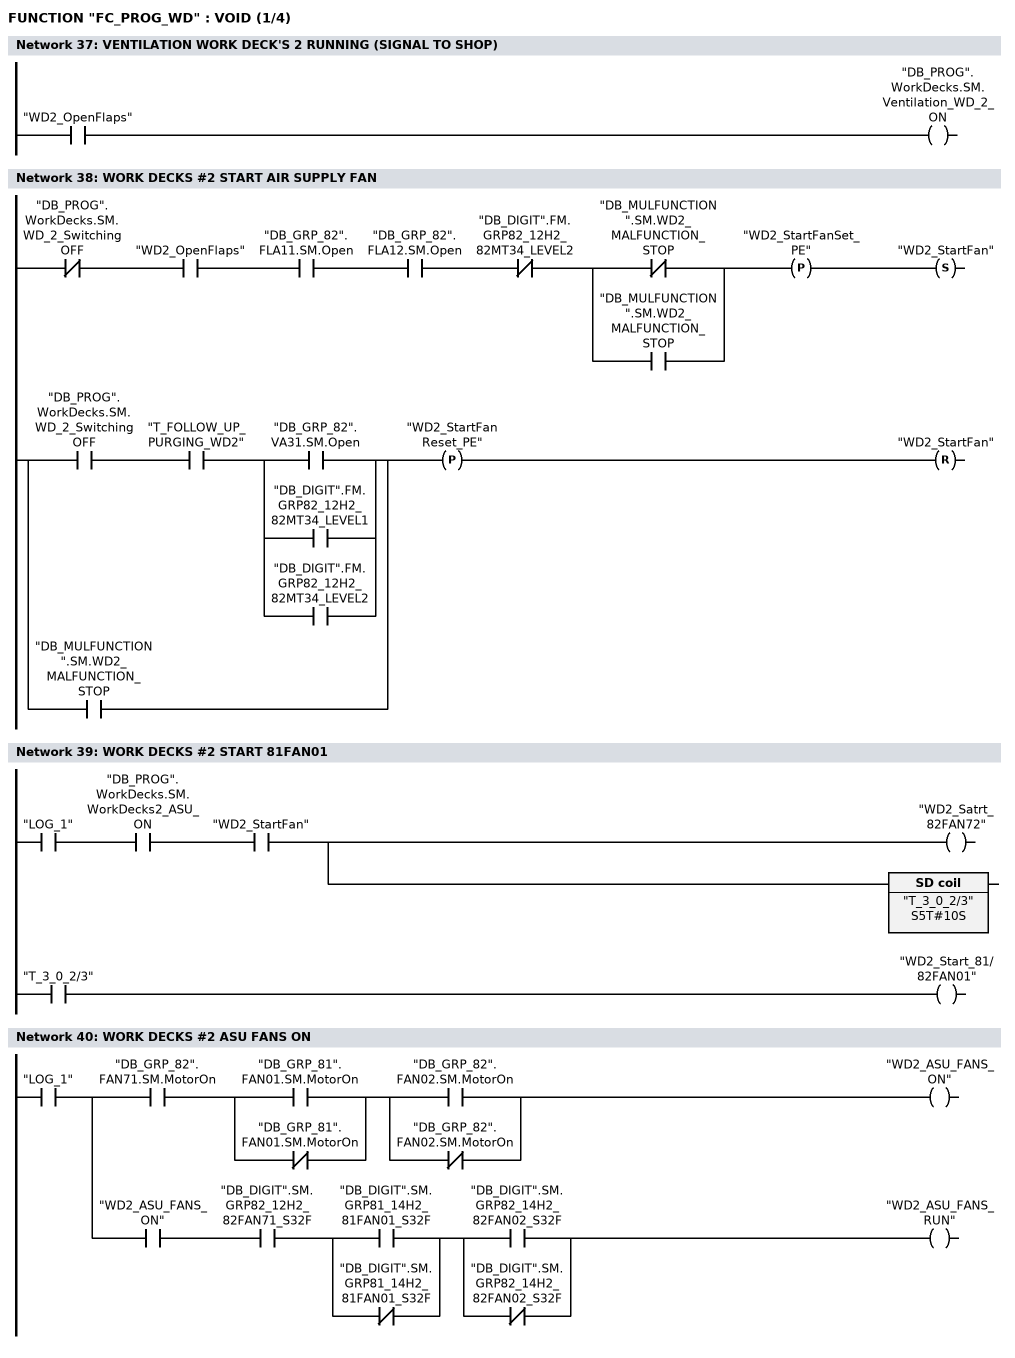
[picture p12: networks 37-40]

      U     "WD2_OpenFlaps";
      =     "DB_PROG".WorkDecks.SM.Ventilation_WD_2_ON;
NETWORK
TITLE =WORK DECKS #2 START AIR SUPPLY FAN

      UN    "DB_PROG".WorkDecks.SM.WD_2_SwitchingOFF;
      U     "WD2_OpenFlaps";
      U     "DB_GRP_82".FLA11.SM.Open;
      U     "DB_GRP_82".FLA12.SM.Open;
      UN    "DB_DIGIT".FM.GRP82_12H2_82MT34_LEVEL2;
      U(    ;
      ON    "DB_MULFUNCTION".SM.WD2_MALFUNCTION_STOP;
      O     "DB_MULFUNCTION".SM.WD2_MALFUNCTION_STOP;
      )     ;
      FP    "WD2_StartFanSet_PE";
      S     "WD2_StartFan";
      U(    ;
      U     "DB_PROG".WorkDecks.SM.WD_2_SwitchingOFF;
      U     "T_FOLLOW_UP_PURGING_WD2";
      U(    ;
      O     "DB_GRP_82".VA31.SM.Open;
      O     "DB_DIGIT".FM.GRP82_12H2_82MT34_LEVEL1;
      O     "DB_DIGIT".FM.GRP82_12H2_82MT34_LEVEL2;
      )     ;
      O     "DB_MULFUNCTION".SM.WD2_MALFUNCTION_STOP;
      )     ;
      FP    "WD2_StartFanReset_PE";
      R     "WD2_StartFan";
      NOP   0;
NETWORK
TITLE =WORK DECKS #2 START 81FAN01

      U     "LOG_1";
      U     "DB_PROG".WorkDecks.SM.WorkDecks2_ASU_ON;
      U     "WD2_StartFan";
      =     L     38.0;
      U     L     38.0;
      BLD   102;
      =     "WD2_Satrt_82FAN72";
      U     L     38.0;
      L     S5T#10S;
      SE    "T_3_0_2/3";
      NOP   0;
      NOP   0;
      NOP   0;
      U     "T_3_0_2/3";
      =     "WD2_Start_81/82FAN01";
NETWORK
TITLE =WORK DECKS #2 ASU FANS ON

      U     "LOG_1";
      =     L     38.0;
      U     L     38.0;
      U     "DB_GRP_82".FAN71.SM.MotorOn;
      U(    ;
      O     "DB_GRP_81".FAN01.SM.MotorOn;
      ON    "DB_GRP_81".FAN01.SM.MotorOn;
      )     ;
      U(    ;
      O     "DB_GRP_82".FAN02.SM.MotorOn;
      ON    "DB_GRP_82".FAN02.SM.MotorOn;
      )     ;
      =     "WD2_ASU_FANS_ON";
      U     L     38.0;
      U     "WD2_ASU_FANS_ON";
      U     "DB_DIGIT".SM.GRP82_12H2_82FAN71_S32F;
      U(    ;
      O     "DB_DIGIT".SM.GRP81_14H2_81FAN01_S32F;
      ON    "DB_DIGIT".SM.GRP81_14H2_81FAN01_S32F;
      )     ;
      U(    ;
      O     "DB_DIGIT".SM.GRP82_14H2_82FAN02_S32F;
      ON    "DB_DIGIT".SM.GRP82_14H2_82FAN02_S32F;
      )     ;
      =     "WD2_ASU_FANS_RUN";
NETWORK
TITLE =WORK DECKS #1 TEMPERATURE CONTROL ON (PAP 2.5.1)
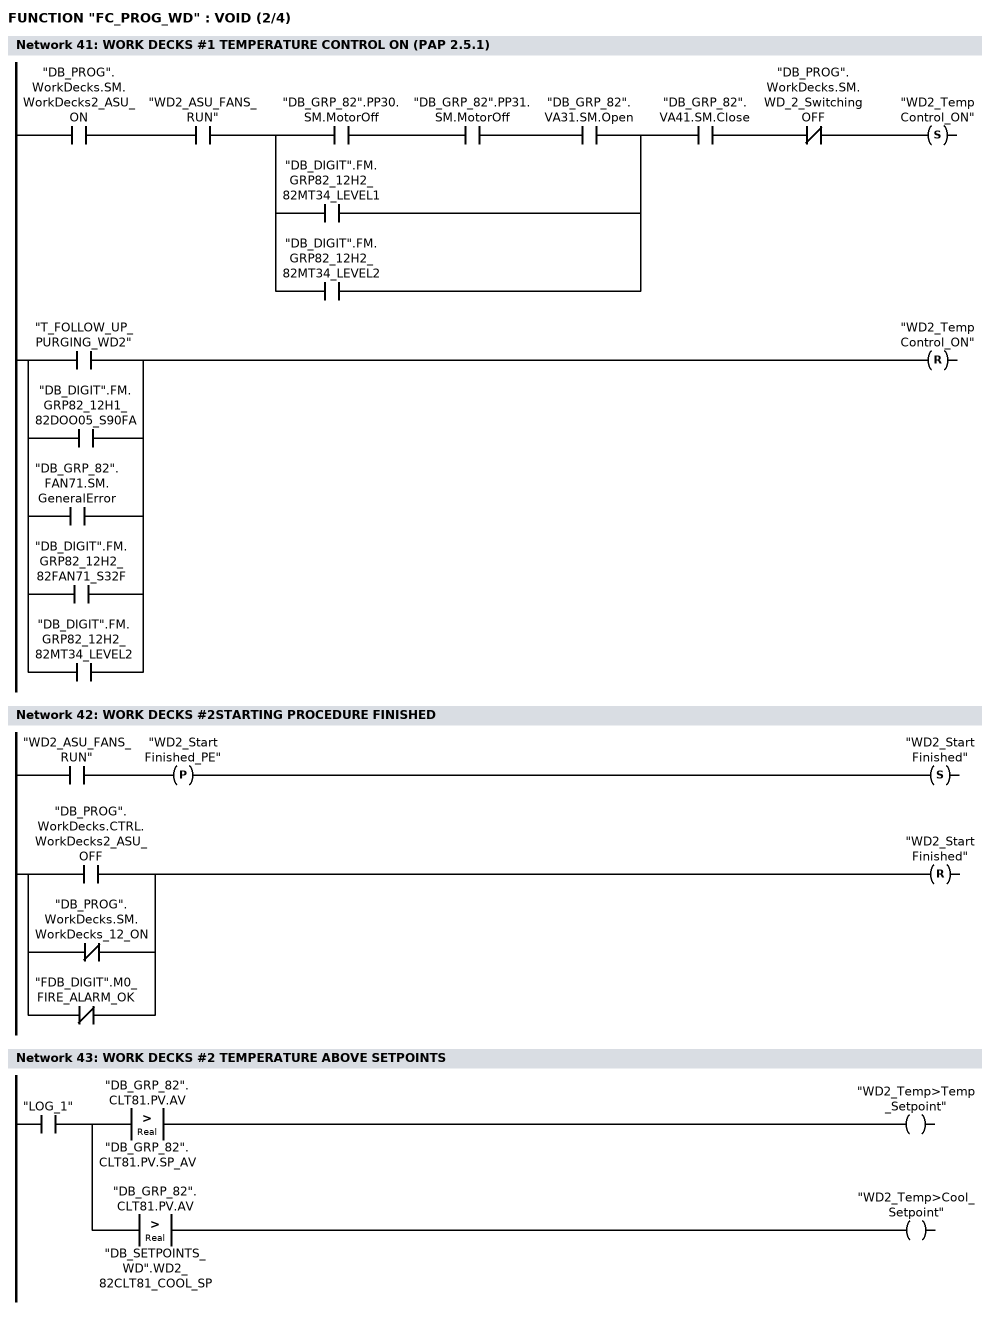
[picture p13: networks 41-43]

      U     "DB_PROG".WorkDecks.SM.WorkDecks2_ASU_ON;
      U     "WD2_ASU_FANS_RUN";
      U(    ;
      U     "DB_GRP_82".PP30.SM.MotorOff;
      U     "DB_GRP_82".PP31.SM.MotorOff;
      U     "DB_GRP_82".VA31.SM.Open;
      O     "DB_DIGIT".FM.GRP82_12H2_82MT34_LEVEL1;
      O     "DB_DIGIT".FM.GRP82_12H2_82MT34_LEVEL2;
      )     ;
      U     "DB_GRP_82".VA41.SM.Close;
      UN    "DB_PROG".WorkDecks.SM.WD_2_SwitchingOFF;
      S     "WD2_TempControl_ON";
      U(    ;
      O     "T_FOLLOW_UP_PURGING_WD2";
      O     "DB_DIGIT".FM.GRP82_12H1_82DOO05_S90FA;
      O     "DB_GRP_82".FAN71.SM.GeneralError;
      O     "DB_DIGIT".FM.GRP82_12H2_82FAN71_S32F;
      O     "DB_DIGIT".FM.GRP82_12H2_82MT34_LEVEL2;
      )     ;
      R     "WD2_TempControl_ON";
      NOP   0;
NETWORK
TITLE =WORK DECKS #2STARTING PROCEDURE FINISHED

      U     "WD2_ASU_FANS_RUN";
      FP    "WD2_StartFinished_PE";
      S     "WD2_StartFinished";
      U(    ;
      O     "DB_PROG".WorkDecks.CTRL.WorkDecks2_ASU_OFF;
      ON    "DB_PROG".WorkDecks.SM.WorkDecks_12_ON;
      ON    "FDB_DIGIT".M0_FIRE_ALARM_OK;
      )     ;
      R     "WD2_StartFinished";
      NOP   0;
NETWORK
TITLE =WORK DECKS #2 TEMPERATURE ABOVE SETPOINTS

      U     "LOG_1";
      =     L     38.0;
      U     L     38.0;
      U(    ;
      L     "DB_GRP_82".CLT81.PV.AV;
      L     "DB_GRP_82".CLT81.PV.SP_AV;
      >R    ;
      )     ;
      =     "WD2_Temp>Temp_Setpoint";
      U     L     38.0;
      U(    ;
      L     "DB_GRP_82".CLT81.PV.AV;
      L     "DB_SETPOINTS_WD".WD2_82CLT81_COOL_SP;
      >R    ;
      )     ;
      =     "WD2_Temp>Cool_Setpoint";
NETWORK
TITLE =WORK DECKS #1 SET SWITCHING POINTS
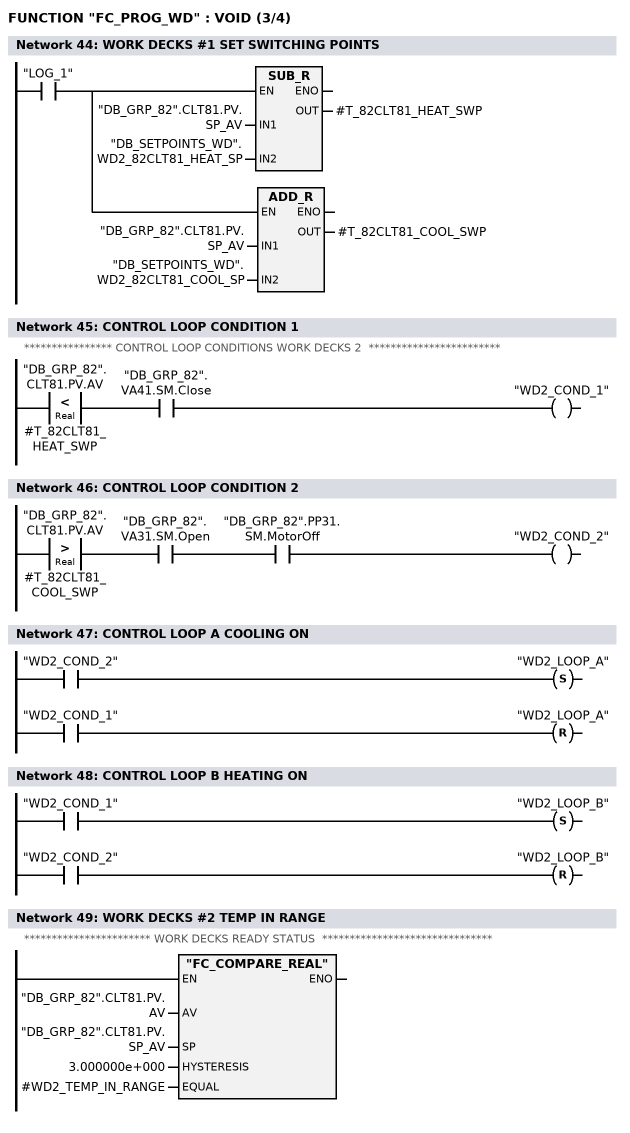
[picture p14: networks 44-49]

      U     "LOG_1";
      =     L     38.0;
      U     L     38.0;
      SPBNB _009;
      L     "DB_GRP_82".CLT81.PV.SP_AV;
      L     "DB_SETPOINTS_WD".WD2_82CLT81_HEAT_SP;
      -R    ;
      T     #T_82CLT81_HEAT_SWP;
_009: NOP   0;
      U     L     38.0;
      SPBNB _00a;
      L     "DB_GRP_82".CLT81.PV.SP_AV;
      L     "DB_SETPOINTS_WD".WD2_82CLT81_COOL_SP;
      +R    ;
      T     #T_82CLT81_COOL_SWP;
_00a: NOP   0;
NETWORK
TITLE =CONTROL LOOP CONDITION 1
//
//**************** CONTROL LOOP CONDITIONS WORK DECKS 2  ************************
//
      U(    ;
      L     "DB_GRP_82".CLT81.PV.AV;
      L     #T_82CLT81_HEAT_SWP;
      <R    ;
      )     ;
      U     "DB_GRP_82".VA41.SM.Close;
      =     "WD2_COND_1";
NETWORK
TITLE =CONTROL LOOP CONDITION 2

      U(    ;
      L     "DB_GRP_82".CLT81.PV.AV;
      L     #T_82CLT81_COOL_SWP;
      >R    ;
      )     ;
      U     "DB_GRP_82".VA31.SM.Open;
      U     "DB_GRP_82".PP31.SM.MotorOff;
      =     "WD2_COND_2";
NETWORK
TITLE =CONTROL LOOP A COOLING ON

      U     "WD2_COND_2";
      S     "WD2_LOOP_A";
      U     "WD2_COND_1";
      R     "WD2_LOOP_A";
      NOP   0;
NETWORK
TITLE =CONTROL LOOP B HEATING ON

      U     "WD2_COND_1";
      S     "WD2_LOOP_B";
      U     "WD2_COND_2";
      R     "WD2_LOOP_B";
      NOP   0;
NETWORK
TITLE =WORK DECKS #2 TEMP IN RANGE
//
//*********************** WORK DECKS READY STATUS  *******************************
//
      CALL "FC_COMPARE_REAL" (
           AV                       := "DB_GRP_82".CLT81.PV.AV,
           SP                       := "DB_GRP_82".CLT81.PV.SP_AV,
           HYSTERESIS               := 3.000000e+000,
           EQUAL                    := #WD2_TEMP_IN_RANGE);
      NOP   0;
NETWORK
TITLE =WORK DECKS #2 WINDOW TO READY STATUS IN POWER SAVING MODE 2
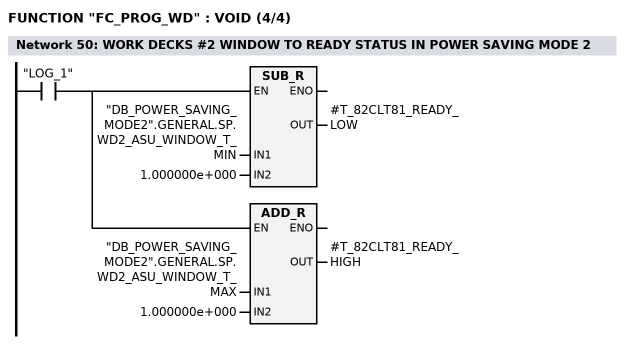
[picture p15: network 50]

      U     "LOG_1";
      =     L     38.0;
      U     L     38.0;
      SPBNB _00b;
      L     "DB_POWER_SAVING_MODE2".GENERAL.SP.WD2_ASU_WINDOW_T_MIN;
      L     1.000000e+000;
      -R    ;
      T     #T_82CLT81_READY_LOW;
_00b: NOP   0;
      U     L     38.0;
      SPBNB _00c;
      L     "DB_POWER_SAVING_MODE2".GENERAL.SP.WD2_ASU_WINDOW_T_MAX;
      L     1.000000e+000;
      +R    ;
      T     #T_82CLT81_READY_HIGH;
_00c: NOP   0;
NETWORK
TITLE =WORK DECKS #2 READY

      U(    ;
      U     "DB_PROG".WorkDecks.SM.WorkDecks2_ASU_ON;
      U(    ;
      O     "DB_PROG".WorkDecks.SM.TimerDone_T_0_0_3;
      O     "DB_PROG".WorkDecks.SM.TimerDone_T_0_0_1;
      )     ;
      U(    ;
      UN    "DB_POWER_SAVING_MODE2".GENERAL.SM.WD2_MODE_2_ON;
      U     #WD2_TEMP_IN_RANGE;
      O     ;
      U     "DB_POWER_SAVING_MODE2".GENERAL.SM.WD2_MODE_2_ON;
      U(    ;
      L     "DB_GRP_82".CLT81.PV.AV;
      L     #T_82CLT81_READY_LOW;
      >=R   ;
      )     ;
      U(    ;
      L     "DB_GRP_82".CLT81.PV.AV;
      L     #T_82CLT81_READY_HIGH;
      <=R   ;
      )     ;
      )     ;
      L     S5T#1M;
      SE    "T_WD2_READY";
      NOP   0;
      NOP   0;
      NOP   0;
      U     "T_WD2_READY";
      )     ;
      S     "DB_PROG".WorkDecks.SM.WD_2_Ready;
      U(    ;
      U(    ;
      ON    "DB_PROG".WorkDecks.SM.WorkDecks2_ASU_ON;
      O     ;
      UN    "DB_POWER_SAVING_MODE2".GENERAL.SM.WD2_MODE_2_ON;
      UN    #WD2_TEMP_IN_RANGE;
      O     ;
      U     "DB_POWER_SAVING_MODE2".GENERAL.SM.WD2_MODE_2_ON;
      U(    ;
      O(    ;
      L     "DB_GRP_82".CLT81.PV.AV;
      L     #T_82CLT81_READY_LOW;
      <R    ;
      )     ;
      O(    ;
      L     "DB_GRP_82".CLT81.PV.AV;
      L     #T_82CLT81_READY_HIGH;
      >R    ;
      )     ;
      )     ;
      )     ;
      L     S5T#1M;
      SE    "T_WD2_READY_LOST_DEL";
      NOP   0;
      NOP   0;
      NOP   0;
      U     "T_WD2_READY_LOST_DEL";
      )     ;
      R     "DB_PROG".WorkDecks.SM.WD_2_Ready;
      NOP   0;
NETWORK
TITLE =END

END_FUNCTION

